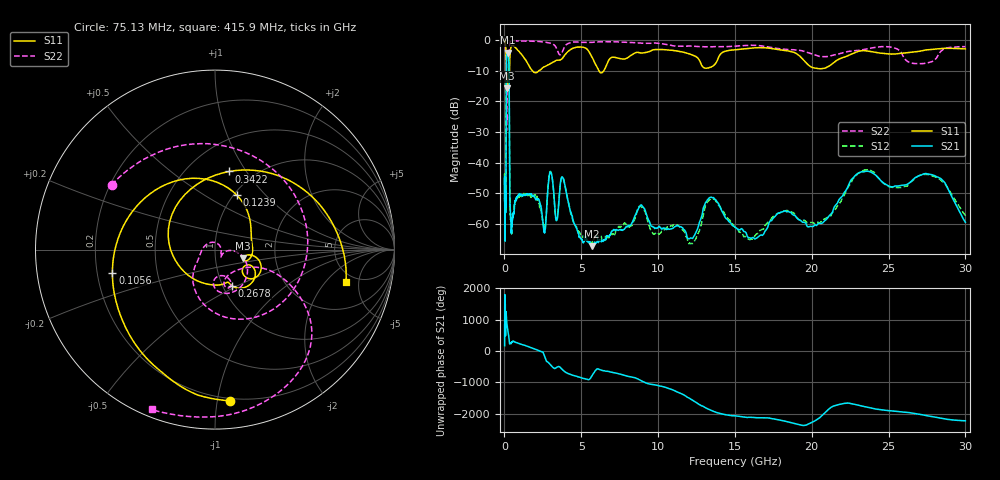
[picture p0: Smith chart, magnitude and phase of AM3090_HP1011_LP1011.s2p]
! Date/Time: Thu, Feb 28, 2019 2:05 PM
! Network Analyzer: Agilent Technologies E8364B Rev: A.07.50.67
! Sweep from 0.010 to 30.000 GHz, 1601 Points, Sweep Type: LOG
! Power Supply: 5.022 V, 0.002 A
# Hz S DB R 50
!freq MagS11 AngS11 MagS21 AngS21 MagS12 AngS12 MagS22 AngS22
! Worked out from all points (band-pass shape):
!   1601 points, 10 MHz to 30 GHz, reference 50 ohm
!   highest |S21| = -4.18 dB at 213.8 MHz (marker M1); lowest = -67.2 dB at 5.697 GHz (marker M2)
!   |S21| within 3 dB of the highest: 131.6 MHz to 288.4 MHz (156.8 MHz wide, 74.7 % of centre)
!   lowest |S11| = -15.7 dB at 159.1 MHz (marker M3), VSWR 1.39, Z = 68.2 - j6.66 ohm
!   |S11| at or under -10 dB: 124.5 MHz to 326.3 MHz (201.8 MHz wide, 89.5 % of centre); 1.811 GHz to 2.24 GHz (428.3 MHz wide, 21.1 % of centre); 6.144 GHz to 6.467 GHz (323.3 MHz wide, 5.13 % of centre)
!   |S22| runs from -29.5 to -0.2 dB; largest |S21 - S12| = 0.011
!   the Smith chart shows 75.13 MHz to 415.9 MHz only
!   S11 on the Smith chart (normalised r, x): 75.13 MHz: 0.18, -1.08; 105.6 MHz: 0.26, -0.10; 123.9 MHz: 1.04, +0.70; 267.8 MHz: 1.10, -0.47; 342.2 MHz: 0.78, +0.84; 415.9 MHz: 4.14, -3.42
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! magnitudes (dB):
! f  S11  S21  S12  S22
! 10 MHz  -0.2  -45.2  -44.8  -0.6
! 38.04 MHz  -0.4  -57.7  -62.2  -1.6
! 75.13 MHz  -1.5  -55.9  -54.9  -3.4
! 105.6 MHz  -4.6  -38.0  -38.0  -5.7
! 123.9 MHz  -9.7  -11.7  -11.6  -13.1
! 144.7 MHz  -13.8  -5.1  -5.1  -25.4
! 159.1 MHz  -15.7  -4.4  -4.4  -22.1
! 213.8 MHz  -14.0  -4.2  -4.1  -14.6
! 267.8 MHz  -13.1  -5.4  -5.4  -13.9
! 303.5 MHz  -14.0  -11.6  -11.5  -8.9
! 342.2 MHz  -7.1  -47.1  -47.3  -1.2
! 415.9 MHz  -2.5  -59.2  -58.0  -0.4
! 550.5 MHz  -1.9  -57.8  -57.2  -0.3
! 2.084 GHz  -10.6  -52.0  -50.8  -0.5
! 2.597 GHz  -8.7  -62.5  -61.8  -0.6
! 2.958 GHz  -7.8  -43.2  -43.0  -1.0
! 3.798 GHz  -5.8  -44.9  -44.6  -3.5
! 5.697 GHz  -5.5  -67.2  -65.9  -0.8
! 7.926 GHz  -6.0  -60.8  -60.4  -0.8
! 16.37 GHz  -2.5  -64.6  -63.3  -1.8
! 23.48 GHz  -3.5  -42.8  -42.4  -3.0
! 30 GHz  -2.9  -59.4  -57.2  -2.2
